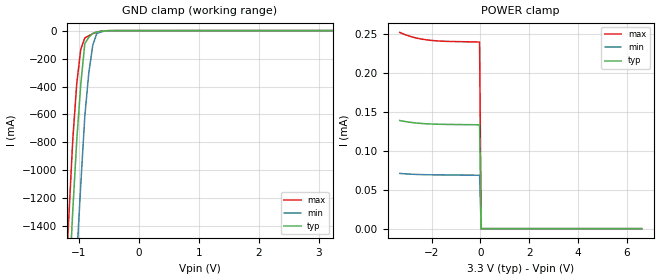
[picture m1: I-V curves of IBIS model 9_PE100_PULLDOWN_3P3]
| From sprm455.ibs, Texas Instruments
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|   Model Cell 9_PE100_PULLDOWN_3P3
|IDG09_PE100_PULLDOWN_3P3
[Model]   9_PE100_PULLDOWN_3P3
Model_type   Input
Polarity   Non-Inverting
Vinl =  0.8V
Vinh =  2V
C_comp   1.604p   1.5372p   1.8937p
[Model Spec]
Vinl   0.8V   0.8V   0.8V
Vinh   2V   2V   2V
[Temperature Range]   25   125   -40
[Voltage Range]   3.3   3   3.6
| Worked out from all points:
|   GND clamp passes 1 mA (typ) near -0.53 V on its own axis
[POWER_clamp]
|   voltage   I(typ)   I(min)   I(max)
-3.3V     139.1uA    71.03uA    252.4uA
-2.7V     136.1uA    69.84uA    245.7uA
-2.1V     134.7uA    69.3uA     242.4uA
-33.33mV  133.5uA    68.69uA    240uA
33.33mV   0A         0A         0A
6.6V      0A         0A         0A
[GND_clamp]
|   voltage   I(typ)   I(min)   I(max)
-3.3V     -22.54A    -23.36A    -22.09A
-1.233V   -2.454A    -3.359A    -1.924A
-1.167V   -1.863A    -2.762A    -1.341A
-1.1V     -1.287A    -2.174A    -780.3mA
-1.033V   -782.3mA   -1.619A    -375.6mA
-966.7mV  -384.2mA   -1.1A      -133mA
-900mV    -93.06mA   -616.1mA   -52.51mA
-833.3mV  -47.65mA   -302.3mA   -36.28mA
-766.7mV  -20.06mA   -103.7mA   -22.29mA
-700mV    -10.32mA   -20.41mA   -10.55mA
-500mV    -344.2uA   -924.1uA   -200.2uA
3.233V    133.5uA    68.76uA    239.7uA
